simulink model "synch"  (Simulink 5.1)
settings: Solver=ode45  StartTime=0.0  StopTime=25.0  RelTol=1e-3
InitFcn:
  | clear functions
libraries: truetime x1, simulink x1

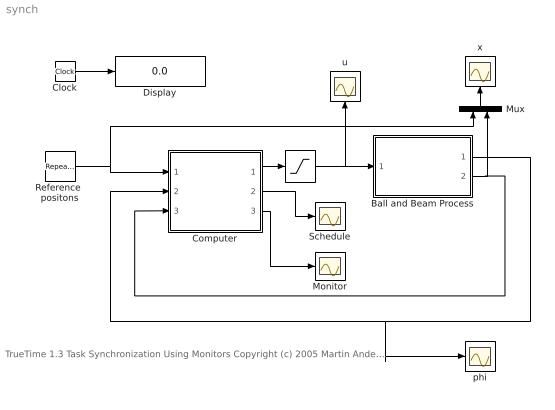
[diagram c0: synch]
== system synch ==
  note: TrueTime 1.3 Task Synchronization Using Monitors Copyright (c) 2005 Martin Andersson, Dan Henriksson and Anton Cervin Department of Automatic Control, Lund University, Sweden Please direct questions and bug reports to: truetime@control.lth.se
  " " : Saturate  UpperLimit=10  LowerLimit=-10  LinearizeAsGain=on
  Ball and Beam Process : Subsystem  SimViewingDevice=off
  Clock : Clock
  Computer : Subsystem  SimViewingDevice=off
  Display : Display
  Monitor : Scope
  Mux : Mux  Orientation=up  Inputs=2
  Reference  positons : simulink/Sources/Repeating Sequence  rep_seq_t=[0 1 1 5 5 9 9 13 13 17 17 21 21 25]  rep_seq_y=[0 0 5 5 -3 -3 8 8 0 0 2 2 -7 -7]
  Schedule : Scope
  phi : Scope
  u : Scope
  x : Scope
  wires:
  Clock/1 -> Display/1
  Ball and Beam Process/2(x) -> Mux/2, Computer/3(AI3)
  Ball and Beam Process/1(phi) -> Computer/2(AI2), phi/1
  Reference  positons/1 -> Computer/1(AI1), Mux/1
  Computer/1(AO1) -> " "/1
  Mux/1 -> x/1
  Computer/2(Schedule) -> Schedule/1
  Computer/3(Monitor) -> Monitor/1
  " "/1 -> u/1, Ball and Beam Process/1(u)

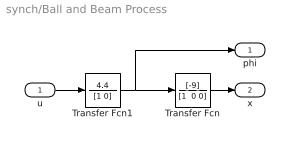
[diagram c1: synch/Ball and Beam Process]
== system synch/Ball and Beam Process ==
  u : Inport  Port=1  PortDimensions=-1  SampleTime=-1  DataType=auto
  Transfer Fcn : TransferFcn  Numerator=[-9]  Denominator="[1  0 0]"  AbsoluteTolerance=auto  Realization=auto
  Transfer Fcn1 : TransferFcn  Numerator=4.4  Denominator=[1 0]  AbsoluteTolerance=auto  Realization=auto
  phi : Outport  Port=1
  x : Outport  Port=2
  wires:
  u/1 -> Transfer Fcn1/1
  Transfer Fcn1/1 -> phi/1, Transfer Fcn/1
  Transfer Fcn/1 -> x/1

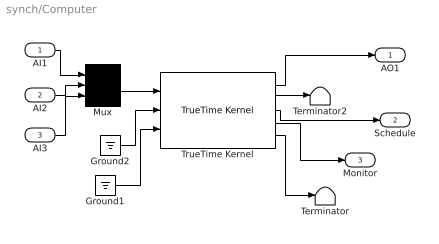
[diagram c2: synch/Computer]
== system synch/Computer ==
  AI1 : Inport  Port=1  PortDimensions=-1  SampleTime=-1  DataType=auto
  AI2 : Inport  Port=2  PortDimensions=-1  SampleTime=-1  DataType=auto
  AI3 : Inport  Port=3  PortDimensions=-1  SampleTime=-1  DataType=auto
  Ground1 : Ground
  Ground2 : Ground
  Mux : Mux  Inputs=3
  Terminator : Terminator
  Terminator2 : Terminator
  TrueTime Kernel : truetime/TrueTime Kernel  sfun=synch_init  args=0  battery=off  clockdrift=0  clockoffset=0
  AO1 : Outport  Port=1
  Schedule : Outport  Port=2
  Monitor : Outport  Port=3
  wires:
  AI1/1 -> Mux/1
  AI2/1 -> Mux/2
  TrueTime Kernel/2 -> Terminator2/1
  Ground2/1 -> TrueTime Kernel/2
  AI3/1 -> Mux/3
  Mux/1 -> TrueTime Kernel/1
  Ground1/1 -> TrueTime Kernel/3
  TrueTime Kernel/4 -> Monitor/1
  TrueTime Kernel/3 -> Schedule/1
  TrueTime Kernel/1 -> AO1/1
  TrueTime Kernel/5 -> Terminator/1
